(* Logix 5000 AddOnInstructionDefinition export AKD_Get_Attribute; software revision 19.01 *)

TYPE AKD_Status :   // All connections to the drive ethernet module are established and data is successfully transferring.
STRUCT
   Profile_In_Progress : BOOL;   // Profile Move In Progress
   Block_In_Execution : BOOL;   // Block In Execution
   On_Target_Position : BOOL;   // On Target Position (1=Current Position Equals Last Target Position)
   General_Fault : BOOL;   // General Fault
   Current_Direction : BOOL;   // Current Motor Direction (0=Reverse, 1=Forward)
   Home_Level : BOOL;   // Level of Home Input
   Reg_Level : BOOL;   // Level of Registration Input
   Enable : BOOL;   // State of Enable Output
   Fault_Input_Fault : BOOL;   // Fault Input Active
   Fwd_Limit : BOOL;   // Forward Input Active
   Rev_Limit : BOOL;   // Reverse Input Active
   Positive_Limit : BOOL;   // Positive Software Limit Exceeded
   Negative_Limit : BOOL;   // Negative Software Limit Exceeded
   FE_Fault : BOOL;   // Following Error Fault
   Block_Fault : BOOL;   // Block Execution Fault
   Load_Complete : BOOL;   // Command Message Successfully Loaded
END_STRUCT
END_TYPE

TYPE AKD_Axis :   // Axis Data:
STRUCT
   Control : AKD_Control;   // Control bits to send to the drive
   Status : AKD_Status;   // Status bits received from the drive
   Input : AB:ETHERNET_MODULE_SINT_64Bytes:I:0;   // Data from the drive
   Output : AB:ETHERNET_MODULE_SINT_64Bytes:O:0;   // Data to the drive
   ResponseMsgType : SINT;   // Response type contained in latest IO response from drive. Used to check for errors
   CommandTimeout : INT;   // Time to allow for command response from drive. Dependent on scan rate and communicaiton rate
   PositionFeedback : DINT;   // Actual Position Value
   VelocityFeedback : DINT;   // Actual Velocity Value
END_STRUCT
END_TYPE

TYPE AKD_Control :   // Send Explicit Message
STRUCT
   Load_Data_Start_Profile : BOOL;   // Load Command Data / Start Profile Move
   Start_Block : BOOL;   // Execute Command block or block chain
   Incremental : BOOL;   // Incremental Position (0=Absolute, 1=Incremental)
   Direction : BOOL;   // Direction in Velocity Mode (0=Reverse, 1=Forward)
   Smooth_Stop : BOOL;   // Smooth / Controlled Stop w/ Deceleration
   Hard_Stop : BOOL;   // Hard / Immediate Stop
   Reg_Arm : BOOL;   // Arm the Registration Input
   Enable : BOOL;   // Enable Output
END_STRUCT
END_TYPE

ADD_ON_INSTRUCTION AKD_Get_Attribute   (* revision 2.1, ExecutePrescan, ExecuteEnableInFalse *)
// Get Position Controller Attribute
// Revision note:
// Don't error if Command_Timeout preset is 0
VAR_OUTPUT
   DN : BOOL; {access Read Only, visible}   // Command Successful
   ER : BOOL; {access Read Only, visible}   // Error
END_VAR
VAR_IN_OUT
   Axis : AKD_Axis; {required}
END_VAR
VAR_INPUT
   Attribute_Number : INT; {visible}   // Attribute Number (see help for options)
END_VAR
VAR_OUTPUT
   Attribute_Value : DINT; {access Read Only, required}   // Attribute Value
END_VAR
VAR
   Command_Timeout : TIMER := (PRE := 100);   // Timeout Timer
   OS_LoadStart : BOOL;
   ErrorSource : SINT;
END_VAR

ROUTINE EnableInFalse   (* ladder *)
// EnableIn_False
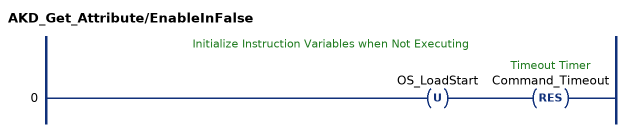
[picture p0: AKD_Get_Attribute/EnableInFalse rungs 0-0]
   // Initialize Instruction Variables when Not Executing
   0: OTU(OS_LoadStart)RES(Command_Timeout);
END_ROUTINE

ROUTINE Logic   (* ladder *)
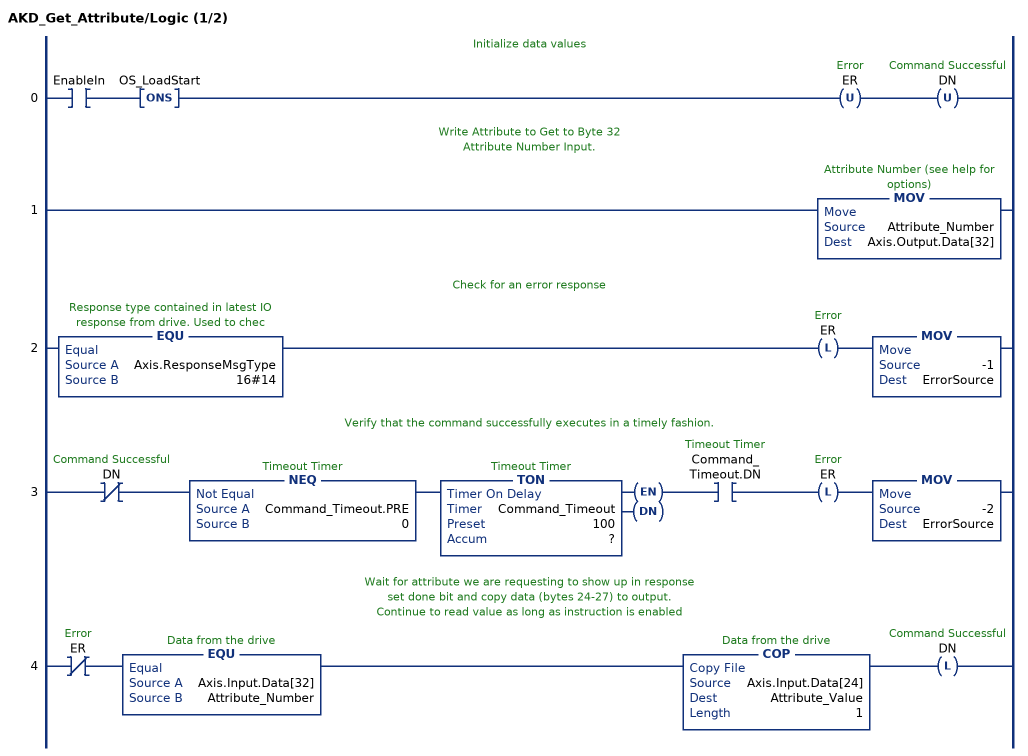
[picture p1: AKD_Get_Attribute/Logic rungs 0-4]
   // Initialize data values
   0: XIC(EnableIn)ONS(OS_LoadStart)OTU(ER)OTU(DN);
   // Write Attribute to Get to Byte 32
   // Attribute Number Input.
   1: MOV(Attribute_Number,Axis.Output.Data[32]);
   // Check for an error response
   2: EQU(Axis.ResponseMsgType,16#14)OTL(ER)MOV(-1,ErrorSource);
   // Verify that the command successfully executes in a timely fashion.
   3: XIO(DN)NEQ(Command_Timeout.PRE,0)TON(Command_Timeout,?,?)XIC(Command_Timeout.DN)OTL(ER)MOV(-2,ErrorSource);
   // Wait for attribute we are requesting to show up in response
   // set done bit and copy data (bytes 24-27) to output.
   // Continue to read value as long as instruction is enabled
   4: XIO(ER)EQU(Axis.Input.Data[32],Attribute_Number)COP(Axis.Input.Data[24],Attribute_Value,1)OTL(DN);
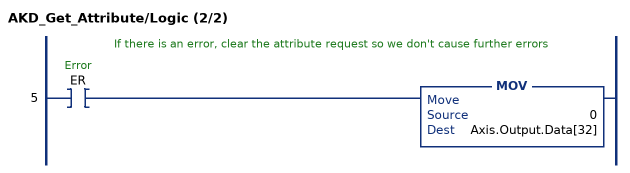
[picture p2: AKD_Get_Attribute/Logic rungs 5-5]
   // If there is an error, clear the attribute request so we don't cause further errors
   5: XIC(ER)MOV(0,Axis.Output.Data[32]);
END_ROUTINE

ROUTINE Prescan   (* ladder *)
// Prescan
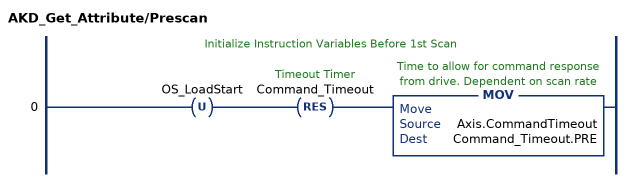
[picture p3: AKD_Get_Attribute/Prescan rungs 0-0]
   // Initialize Instruction Variables Before 1st Scan
   0: OTU(OS_LoadStart)RES(Command_Timeout)MOV(Axis.CommandTimeout,Command_Timeout.PRE);
END_ROUTINE
END_ADD_ON_INSTRUCTION
